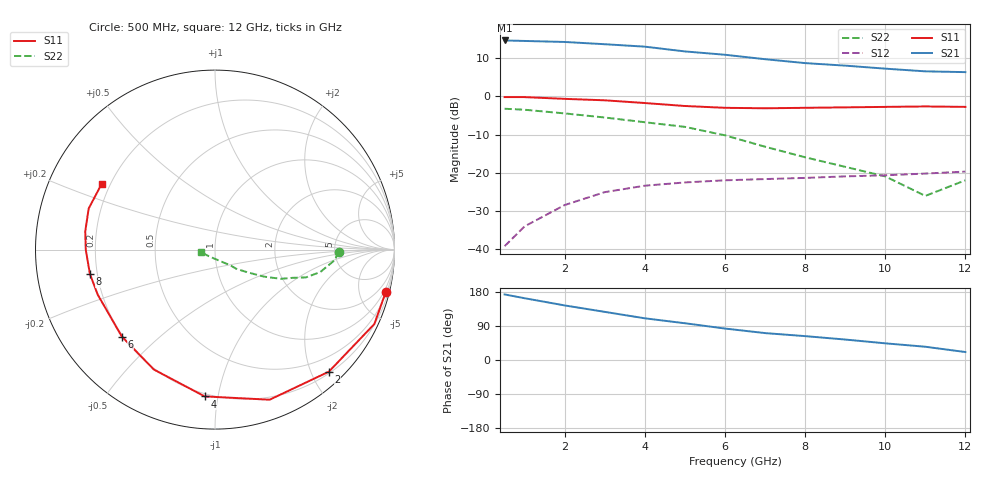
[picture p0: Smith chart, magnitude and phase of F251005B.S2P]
!ATF-25100
!S-PARAMETERS at Vds=5V  Id=50mA.  LAST UPDATED 07-22-92
# ghz s ma r 50
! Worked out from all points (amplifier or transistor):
!   13 points, 500 MHz to 12 GHz, reference 50 ohm
!   highest |S21| = 14.6 dB at 500 MHz (marker M1)
!   |S21| within 3 dB of that: start of sweep to 5.148 GHz
!   unconditionally stable (mu >= 1): 7.157 GHz to end of sweep
!   at 2 GHz: K = 0.28, MSG = 21.3 dB, |S12| = -28.4 dB
!   at 6 GHz: K = 0.85, MSG = 16.4 dB, |S12| = -21.9 dB
!   at 12 GHz: K = 1.17, MAG = 10.5 dB, |S12| = -19.7 dB
!   S11 on the Smith chart (normalised r, x): 500 MHz: 0.68, -8.09; 2 GHz: 0.23, -2.28; 4 GHz: 0.18, -0.92; 6 GHz: 0.20, -0.38; 8 GHz: 0.17, -0.09; 12 GHz: 0.17, +0.26
0.5  0.98 -14.0  5.4 173.0  0.011 88.0  0.69 -1.0
1  0.98 -25.0  5.32 163.0  0.02 82.0  0.67 -5.0
2  0.93 -47.0  5.16 144.0  0.038 71.0  0.6 -12.0
3  0.89 -70.0  4.82 127.0  0.056 65.0  0.53 -17.0
4  0.82 -94.0  4.48 110.0  0.068 52.0  0.46 -20.0
5  0.75 -117.0  3.88 97.0  0.075 50.0  0.4 -24.0
6  0.71 -137.0  3.51 83.0  0.08 46.0  0.31 -29.0
7  0.7 -159.0  3.07 71.0  0.083 42.0  0.22 -35.0
8  0.71 -169.0  2.73 63.0  0.086 41.0  0.16 -42.0
9  0.72 180.0  2.53 54.0  0.09 40.0  0.12 -46.0
10  0.73 172.0  2.31 44.0  0.093 39.0  0.09 -55.0
11  0.74 162.0  2.13 35.0  0.098 36.0  0.05 -131.0
12  0.73 150.0  2.08 21.0  0.104 34.0  0.08 -170.0
